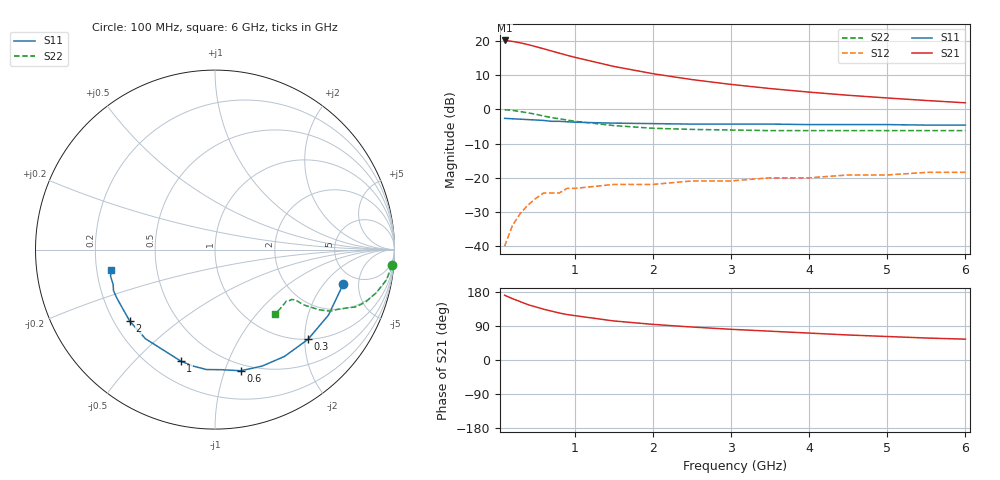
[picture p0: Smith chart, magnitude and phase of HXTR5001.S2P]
! HXTR-5001 Common Emitter
! Vce=18V  Ic=30mA
# ghz s ma r 50
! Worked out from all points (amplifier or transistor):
!   20 points, 100 MHz to 6 GHz, reference 50 ohm
!   highest |S21| = 20.2 dB at 100 MHz (marker M1)
!   |S21| within 3 dB of that: start of sweep to 688.5 MHz
!   unconditionally stable (mu >= 1): 2.83 GHz to end of sweep
!   at 400 MHz: K = 0.16, MSG = 23.5 dB, |S12| = -28.0 dB
!   at 1.5 GHz: K = 0.58, MSG = 17.3 dB, |S12| = -21.9 dB
!   at 6 GHz: K = 1.54, MAG = 5.9 dB, |S12| = -18.4 dB
!   S11 on the Smith chart (normalised r, x): 100 MHz: 3.83, -3.25; 300 MHz: 1.00, -2.07; 600 MHz: 0.44, -1.14; 1 GHz: 0.32, -0.69; 2 GHz: 0.26, -0.34; 6 GHz: 0.26, -0.09
0.1  0.74 -15.0  10.2 171.0  0.01 83.0  0.99 -5.0
0.2  0.73 -30.0  9.88 162.0  0.02 75.0  0.97 -10.0
0.3  0.72 -44.0  9.42 154.0  0.03 69.0  0.93 -15.0
0.4  0.71 -57.0  8.87 146.0  0.04 63.0  0.89 -19.0
0.5  0.7 -68.0  8.28 140.0  0.05 58.0  0.85 -22.0
0.6  0.69 -78.0  7.71 134.0  0.06 54.0  0.8 -24.0
0.7  0.67 -87.0  7.16 129.0  0.06 50.0  0.76 -26.0
0.8  0.67 -94.0  6.65 124.0  0.06 47.0  0.73 -28.0
0.9  0.66 -101.0  6.19 120.0  0.07 44.0  0.7 -29.0
1  0.65 -107.0  5.78 117.0  0.07 42.0  0.67 -30.0
1.5  0.63 -128.0  4.25 103.0  0.08 37.0  0.58 -32.0
2  0.62 -140.0  3.33 94.0  0.08 35.0  0.53 -32.0
2.5  0.61 -148.0  2.73 87.0  0.09 35.0  0.51 -33.0
3  0.61 -154.0  2.32 81.0  0.09 35.0  0.5 -35.0
3.5  0.61 -158.0  2.02 76.0  0.1 36.0  0.49 -36.0
4  0.6 -161.0  1.79 71.0  0.1 37.0  0.49 -38.0
4.5  0.6 -164.0  1.61 66.0  0.11 38.0  0.49 -40.0
5  0.6 -166.0  1.47 62.0  0.11 39.0  0.49 -43.0
5.5  0.59 -168.0  1.35 58.0  0.12 40.0  0.49 -45.0
6  0.59 -169.0  1.25 55.0  0.12 40.0  0.49 -47.0
